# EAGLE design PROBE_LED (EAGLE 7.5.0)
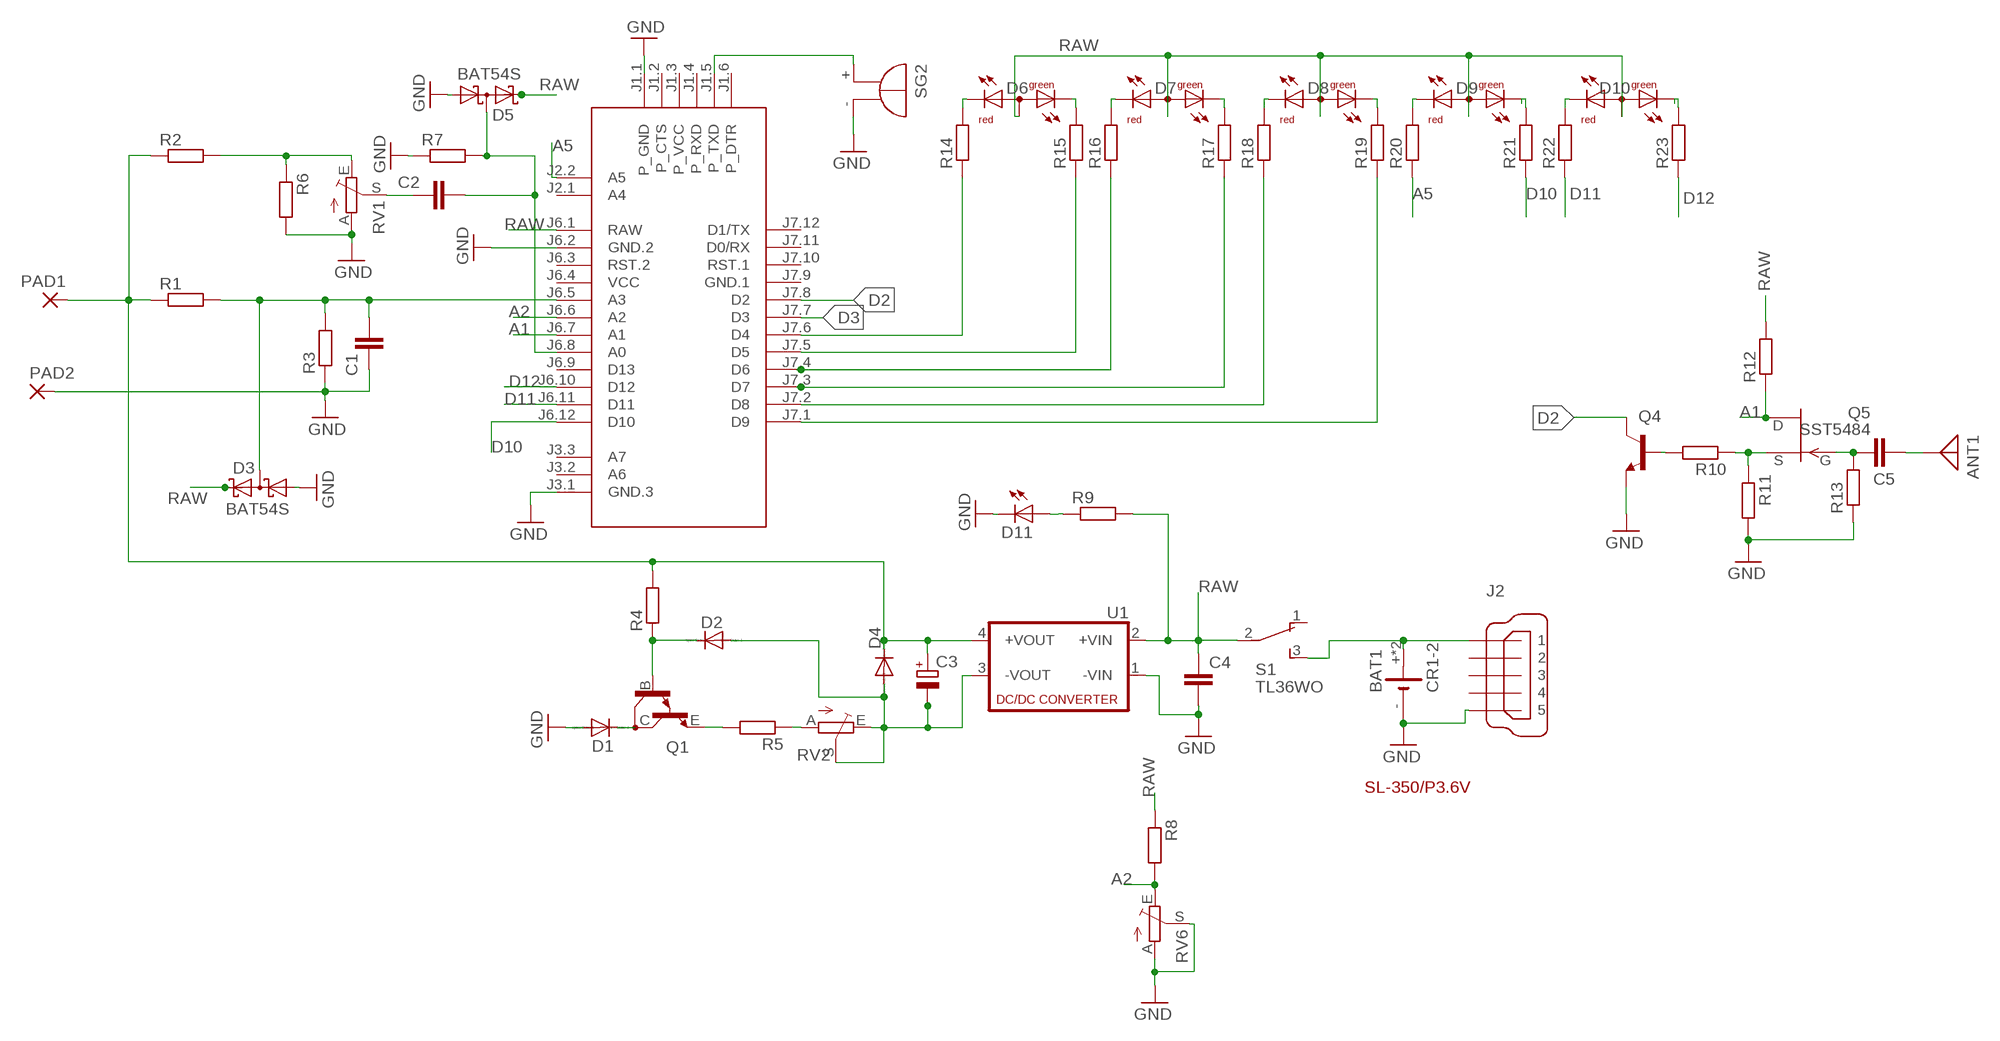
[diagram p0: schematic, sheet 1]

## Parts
ANT1  ANTENNA  [PAD-01]
ARD1  ARDUINO-PRO-MINI-3.3V  [ARDUINO-PRO-MINI]
BAT1  CR1-2  [CR1-2]
C1  C-EUC1206  [C1206]
C2  C-EUC1206  [C1206]
C3  CPOL-EUC/6032-28R  [C/6032-28R]
C4  C-EUC1206  [C1206]
C5  C-EUC1206  [C1206]
D1  CGRM4007-G  [SOD-123_MINI-SMA]
D2  CGRM4007-G  [SOD-123_MINI-SMA]
D3  BAT54S  [SOT23]
D4  CGRM4001-G  [SOD-123_MINI-SMA]
D5  BAT54S  [SOT23]
D6  DUOLED-RG-A  [DUOLED-A-5MM]
D7  DUOLED-RG-A  [DUOLED-A-5MM]
D8  DUOLED-RG-A  [DUOLED-A-5MM]
D9  DUOLED-RG-A  [DUOLED-A-5MM]
D10  DUOLED-RG-A  [DUOLED-A-5MM]
D11  LED5MM  [LED5MM]
J2  MINI-USB_SHIELD5P2-32005-601  [32005-601]
PAD1  3,81/1,1  [3,81/1,1]
PAD2  3,81/1,1  [3,81/1,1]
Q1  BDV65  [SOT93]
Q4  BC817-16LT1SMD  [SOT23-BEC]
Q5  SST5484  [SOT23]
R1  R-EU_R2512  [R2512]
R2  R-EU_R2512  [R2512]
R3  R-EU_R2512  [R2512]
R4  R-EU_R2512  [R2512]
R5  R-EU_R2512  [R2512]
R6  R-EU_R2512  [R2512]
R7  R-EU_R0805  [R0805]
R8  R-EU_R0805  [R0805]
R9  R-EU_R0805  [R0805]
R10  R-EU_R0805  [R0805]
R11  R-EU_R0805  [R0805]
R12  R-EU_R1206  [R1206]
R13  R-EU_R0805  [R0805]
R14  R-EU_R0805  [R0805]
R15  R-EU_R0805  [R0805]
R16  R-EU_R0805  [R0805]
R17  R-EU_R0805  [R0805]
R18  R-EU_R0805  [R0805]
R19  R-EU_R0805  [R0805]
R20  R-EU_R0805  [R0805]
R21  R-EU_R0805  [R0805]
R22  R-EU_R0805  [R0805]
R23  R-EU_R0805  [R0805]
RV1  TRIM_EU-CT6  [CT6]
RV2  TRIM_EU-CT6  [CT6]
RV6  TRIM_EU-CT6  [CT6]
S1  TL36WO  [TL3XWO]
SG2  BMT1205XH7.5  [BMT1205XH7.5]
U1  NME  [NME]

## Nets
A1: ARD1.J6.7(A1) Q5.2(D) R12.1
A2: ARD1.J6.6(A2) R8.2 RV6.E
A3: ARD1.J6.5(A3) C1.2 D3.3(C1A2) R1.2 R3.2
A5: ARD1.J2.2(A5) R20.1
D2: ARD1.J7.8(D2) Q4.C
D3: ARD1.J7.7(D3)
D10: ARD1.J6.12(D10) R21.1
D11: ARD1.J6.11(D11) R22.1
D12: ARD1.J6.10(D12) R23.1
GND: ARD1.J1.1(P_GND) ARD1.J3.1(GND.3) ARD1.J6.2(GND.2) BAT1.- C1.1 C4.2 D1.A D3.1(A1) D5.1(A1) D11.K(C) J2.5 PAD2.1(P) Q4.E R3.1 R6.2 R7.1 R11.2 R13.1 RV1.A RV6.A RV6.S SG2.- U1.1(-VIN)
N$1: R2.2 R6.1 RV1.E
N$2: Q4.B R10.2
N$3: Q5.3(S) R10.1 R11.1
N$4: ARD1.J6.8(A0) C2.2 D5.3(C1A2) R7.2
N$5: ARD1.J1.5(P_TXD) SG2.+
N$6: BAT1.+ BAT1.+@1(+) J2.1 S1.3(S)
N$7: ANT1.1 C5.2
N$8: Q1.E R5.2
N$9: R5.1 RV2.A
N$10: C3.- D2.A D4.A RV2.E RV2.S U1.3(-VOUT)
N$11: D6.CR R14.2
N$12: D1.C Q1.C
N$13: C5.1 Q5.1(G) R13.2
N$14: D6.CX(CG) R15.2
N$15: D7.CR R16.2
N$16: D7.CX(CG) R17.2
N$17: D8.CR R18.2
N$18: D8.CX(CG) R19.2
N$19: D9.CR R20.2
N$20: D2.C Q1.B R4.1
N$21: D9.CX(CG) R21.2
N$22: D10.CR R22.2
N$23: C2.1 RV1.S
N$24: C3.+ D4.C PAD1.1(P) R1.1 R2.1 R4.2 U1.4(+VOUT)
N$25: D10.CX(CG) R23.2
N$26: ARD1.J7.6(D4) R14.1
N$27: ARD1.J7.5(D5) R15.1
N$28: ARD1.J7.4(D6) R16.1
N$29: ARD1.J7.3(D7) R17.1
N$30: ARD1.J7.2(D8) R18.1
N$31: ARD1.J7.1(D9) R19.1
N$32: D11.A R9.1
RAW: ARD1.J6.1(RAW) C4.1 D3.2(C2) D5.2(C2) D6.A D7.A D8.A D9.A D10.A R8.1 R9.2 R12.2 S1.2(P) U1.2(+VIN)
Unconnected: ARD1.J1.2(P_CTS) ARD1.J1.3(P_VCC) ARD1.J1.4(P_RXD) ARD1.J1.6(P_DTR) ARD1.J2.1(A4) ARD1.J3.2(A6) ARD1.J3.3(A7) ARD1.J6.3(RST.2) ARD1.J6.9(D13) ARD1.J7.10(RST.1) ARD1.J7.11(D0/RX) ARD1.J7.12(D1/TX) J2.2 J2.3 J2.4 J2.M1(S1) J2.M2(S2) S1.1(O)

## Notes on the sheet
- SL-350/P3.6V

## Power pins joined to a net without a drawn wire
GND.1: ARD1.J7.9(GND.1)
VCC: ARD1.J6.4(VCC)

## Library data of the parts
ANT1 = discrete:ANTENNA: Antenna
ARD1 = diy-modules:ARDUINO-PRO-MINI-*: Arduino Pro Mini and compatible devices More details available here: https://www.arduino.cc/en/Main/ArduinoBoardProMini Click here to find device on ebay.com
BAT1 = battery:CR1-2
C1 C2 C4 C5 = rcl:C-EU: CAPACITOR, European symbol
C3 = rcl:CPOL-EU: POLARIZED CAPACITOR, European symbol
D1 D2 D4 = diode:CGRM400*-G: Molded plasitc,JEDEC SOD-123/Mini SMA
D3 D5 = diode:BAT54S: Schottky Diodes Pin connection corrected 2011-05-04 Source: Fairchild .. BAT54.pdf
D6-D10 = led:DUOLED-RG-A: DUO LED 2 colors (red/green), 5 mm, round, common Anode www.ligitek.com or other producers.
D11 = led:LED: LED
J2 = con-cypressindustries:MINI-USB_SHIELD5P2-: MINI USB-B R/A DIP 5pol. Source: www.cypressindustries.com; OC_FARNELL: unknown; OC_NEWARK: unknown
PAD1 PAD2 = wirepad:3,81/1,1: THROUGH-HOLE PAD
Q1 = transistor:BDV65: NPN BIPOLAR DARLINGTON TRANSISTOR
Q4 = transistor-npn:BC817*: NPN Transistor
Q5 = transistor-fet:?548*: N-Channel JFETs Source: VISHAY 2N5484.pdf Compatible: TO92 2N5245 J304 J305 U310 J308 J309 J310 TO72 2N4416 2N4416A 2N3823 2N4351 3N169 3N170 3N171 MFE3002 TO18 2N3796 2N3797 MFE825 Source: Motorola European Master Guide Pacge 3-59
R1-R23 = rcl:R-EU_: RESISTOR, European symbol
RV1 RV2 RV6 = pot:TRIM_EU-: POTENTIOMETER
S1 = switch:TL36WO: TINY SWITCH ON - ON Source: http://www2.produktinfo.conrad.com/datenblaetter/700000-724999/705152-da-01-de-Subminiaturschalter_TL_36WO.pdf
SG2 = buzzer:BMT1205XH7.5: MAGNETIC TRANSDUCER; OC_FARNELL: unknown; OC_NEWARK: unknown
U1 = dc-dc-converter:NME: DC-DC CONVERTER; MF: C & D TECHNOLOGIES, INC; MPN: NME1205D; OC_FARNELL: 1021466; OC_NEWARK: 98B8198

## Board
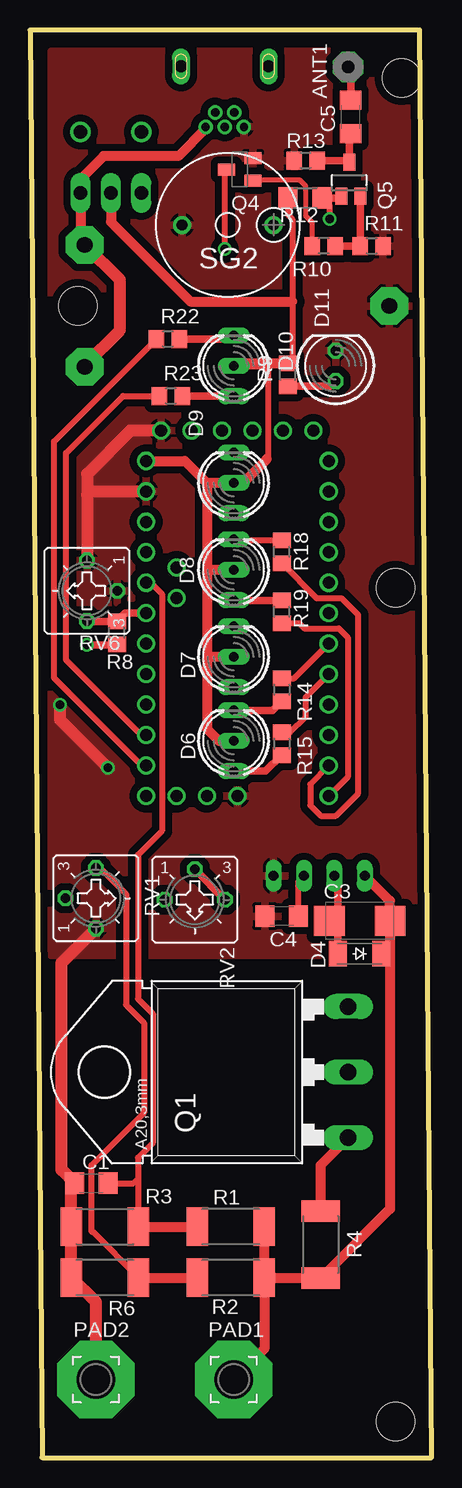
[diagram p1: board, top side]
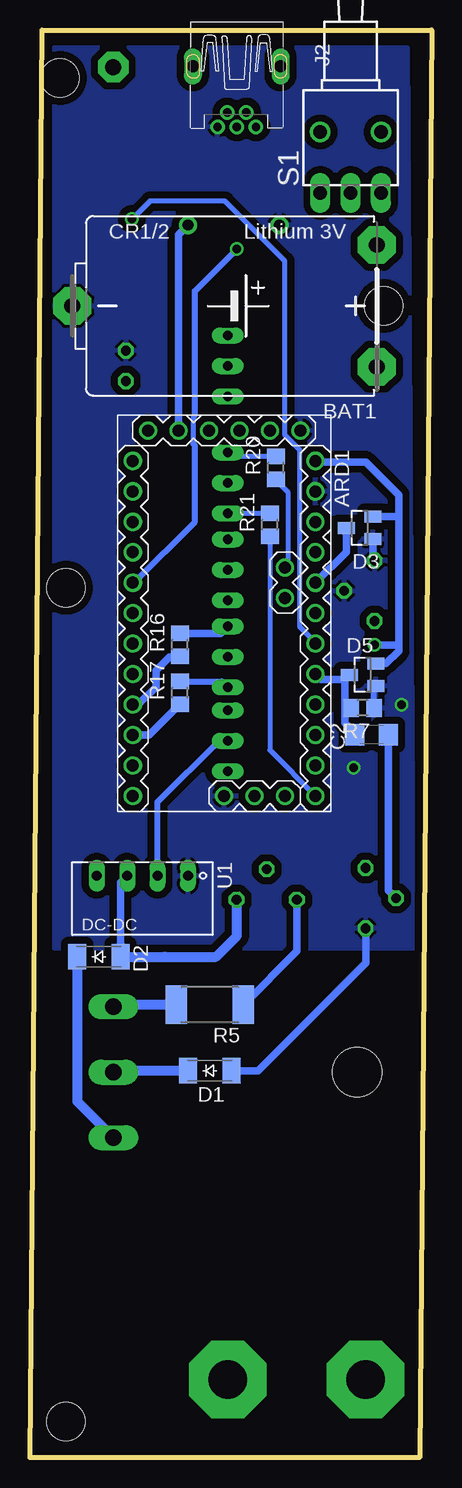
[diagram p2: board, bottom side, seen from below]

Size 33.5 x 119 mm. Coordinates in mm from the lower left corner, seen from the top.
Outline: 1,0 33.5,0 32.5,119 0,119 1,0
Copper layers (1*16): Top 0.035mm / dielectric 1.5mm / Bottom 0.035mm
Design rules "default *": minimum track width 10mil, minimum drill 24mil, track to track 8mil, track to pad 8mil, pad to pad 8mil, via to via 8mil, smd to smd 8mil, copper to edge 20mil, drill to drill 8mil, minimum pad ring 10mil, minimum via ring 8mil, stop-mask expansion 4mil, vias tented up to drill 0mil, thermal gap 10mil
Holes 3.2 mm at 31,115 30.5,3 30.5,72.5 4,96
bRestrict: area 1.4,22.6 to 11,28.2

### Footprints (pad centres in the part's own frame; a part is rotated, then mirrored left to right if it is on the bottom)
PAD-01 = drill 1.321 pad 2.54 octagon: 1 0,0
ARDUINO-PRO-MINI = drill 1: J1.1 -15.24,6.35; J1.2 -15.24,3.81; J1.3 -15.24,1.27; J1.4 -15.24,-1.27; J1.5 -15.24,-3.81; J1.6 -15.24,-6.35; J2.1 -1.27,5.08; J2.2 -3.81,5.08; J3.1 15.24,0; J3.2 15.24,2.54; J3.3 15.24,5.08; J6.1 -12.7,7.62; J6.2 -10.16,7.62; J6.3 -7.62,7.62; J6.4 -5.08,7.62; J6.5 -2.54,7.62; J6.6 0,7.62; J6.7 2.54,7.62; J6.8 5.08,7.62; J6.9 7.62,7.62; J6.10 10.16,7.62; J6.11 12.7,7.62; J6.12 15.24,7.62; J7.1 15.24,-7.62; J7.2 12.7,-7.62; J7.3 10.16,-7.62; J7.4 7.62,-7.62; J7.5 5.08,-7.62; J7.6 2.54,-7.62; J7.7 0,-7.62; J7.8 -2.54,-7.62; J7.9 -5.08,-7.62; J7.10 -7.62,-7.62; J7.11 -10.16,-7.62; J7.12 -12.7,-7.62
CR1-2 = drill 1.321 pad 3.15 octagon: + -11.43,-5.08; +@1 -11.43,5.08; - 13.97,0
C1206 = smd 1.6 x 1.8: 1 -1.4,0; 2 1.4,0
C/6032-28R = smd 2.55 x 2.5: + 2.525,0; - -2.525,0
SOD-123_MINI-SMA = smd 1.5 x 2.1: A 1.8,0; C -1.8,0
SOT23 = smd 1 x 1.4: 1 -0.95,-1.1; 2 0.95,-1.1; 3 0,1.1
DUOLED-A-5MM = drill 0.813 long: A 0,0; CR 2.54,0; CX -2.54,0
LED5MM = drill 0.813 octagon: A -1.27,0; K 1.27,0
32005-601 = drill 0.7 pad 1.016: 1 2.825,1.6; 2 1.625,0.8; 3 2.825,0; 4 1.625,-0.8; 5 2.825,-1.6 | drill 1 pad 1.422 long: M1 -2.225,3.65; M2 -2.225,-3.65
3,81/1,1 = drill 3.2 pad 6.452 octagon: 1 0,0
SOT93 = drill 1.397 long: B -5.461,-10.16; C 0,-10.16; E 5.461,-10.16 | hole 4.115: 0,10.16
SOT23-BEC = smd 1 x 1.4: B -0.95,-1.1; C 0,1.1; E 0.95,-1.1
SOT23' = smd 1 x 1.4: 1 0,1.735; 2 -0.632,-1.1; 3 0.95,-1.1
R2512 = smd 1.8 x 3.2: 1 -2.8,0; 2 2.8,0
R0805 = smd 1.3 x 1.5: 1 -0.95,0; 2 0.95,0
R1206 = smd 1.6 x 1.803: 1 -1.422,0; 2 1.422,0
CT6 = drill 0.813 octagon: A 2.515,0; E -2.515,0; S 0,-2.54
TL3XWO = drill 1.1 pad 1.422 long: 1 -2.54,-5.08; 2 0,-5.08; 3 2.54,-5.08 | drill 1.1 pad 1.676: M1 -2.54,0; M2 2.54,0
BMT1205XH7.5 = drill 0.9 pad 1.5: + 3.8,0; - -3.8,0
NME = drill 0.813 long: 1 0,3.81; 2 0,1.27; 3 0,-1.27; 4 0,-3.81

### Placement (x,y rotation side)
ANT1  26.55,115.91 0 top
ARD1  17.3,70.38 270 bottom
BAT1  16,96 180 bottom
C1  5.12,22.88 0 top
C2  5,60.25 180 bottom
C3  27.5,44.75 0 top
C4  21,45.12 180 top
C5  26.75,111.75 90 top
D1  18.5,32.25 0 bottom
D2  27.75,41.75 0 bottom
D3  6,77.5 90 bottom
D4  27.5,42 180 top
D5  5.75,65.25 90 bottom
D6  17,59.75 90 top
D7  17,66.75 90 top
D8  17,74 90 top
D9  17,81.25 90 top
D10  17,91 90 top
D11  25.5,91 90 top
J2  16.25,113.75 270 bottom
PAD1  17,6.5 0 top
PAD2  5.5,6.5 0 top
Q1  16.38,32.12 90 top
Q4  17.5,107.38 90 top
Q5  SST5484  [SOT23']  26.62,106.25 0 top
R1  16.75,19.25 180 top
R2  16.75,15 180 top
R3  6.25,19.25 0 top
R4  24.25,17.75 270 top
R5  18.5,37.75 180 bottom
R6  6.25,15 180 top
R7  5.75,62.5 180 bottom
R8  7.25,68.75 90 top
R9  21.5,90.25 90 top
R10  24.5,101 180 top
R11  28.5,101 0 top
R12  22.95,105 180 top
R13  23,108.12 0 top
R14  21,64 270 top
R15  21,59.5 270 top
R16  21,67.75 90 bottom
R17  21,63.75 90 bottom
R18  21,75.5 90 top
R19  21,70.5 90 top
R20  13,82.5 90 bottom
R21  13.5,77.75 90 bottom
R22  11.5,93.25 0 top
R23  11.75,88.5 0 top
RV1  5.5,46.62 270 top
RV2  13.75,46.5 180 top
RV6  4.75,72.25 90 top
S1  6.75,110.5 0 bottom
SG2  16.5,102.75 0 top
U1  24.12,48.5 270 bottom

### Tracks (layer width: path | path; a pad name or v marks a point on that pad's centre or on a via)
A1  (via drill 0.7)
  Top 0.406: 24.5,104.87 R12.1
  Top 0.5: v25,103.25 25,104.37 R12.1
  Top 0.61: R12.1 25.84,105 Q5.2
  Bottom 0.406: ARD1.J6.7 9.68,67.93 11,69.25 11,84 12.25,85.25 12.25,99.75 17.25,104.75 23.5,104.75 v25,103.25
A2
  Top 0.61: RV6.E 4.79,69.7 R8.2 7.93,70.38 ARD1.J6.6
A3
  Top 0.5: 9,23.25 9,25 10.25,26.25 10.25,37 9,38.25 9,50.25 11,52.25 11,72 10.08,72.92 ARD1.J6.5 | 9,23.25 9,19.3 R3.2 | C1.2 8.62,22.88 9,23.25
  Top 0.813: R3.2 R1.2
  Bottom 0.61: D3.3 7.1,75.5 ARD1.J6.5
A5
  Bottom 0.406: R20.1 13,81.5 12,80.5 12,74.41 ARD1.J2.2
D2  (via drill 0.7)
  Top 0.5: v16.25,100.75 16.25,107.22 Q4.C
  Bottom 0.406: 19.88,84.5 19.88,86.75 19.75,86.88
  Bottom 0.5: ARD1.J7.8 24.83,72.92 19.75,78 19.75,84.38 19.88,84.5 | v16.25,100.75 19.75,97.25 19.75,86.88
D10
  Bottom 0.406: R21.1 13.5,58.96 ARD1.J6.12
D11
  Top 0.5: ARD1.J6.11 9.32,57.68 2,65 2,84.7 R22.1
D12
  Top 0.5: ARD1.J6.10 9.28,60.22 3,66.5 3,83.75 7.75,88.5 R23.1
GND  (via drill 0.7)
  Top 1.016: RV1.A 2.62,41.23 2.62,23.98 C1.1 3.45,22.6 R3.1 R6.2 5.5,12.95 PAD2.1 | v6.5,57.5 2.5,61.5 v2.5,62.75 | ARD1.J1.1 8.37,85.62 4.75,82 4.75,80.25 | 4.75,80.25 RV6.A | ARD1.J6.2 5.04,80.54 4.75,80.25
  Bottom 0.5: R7.1 4.8,64.15 D5.1
  Bottom 0.61: D3.1 4.9,74.92 RV6.A | D1.A 14.5,32.25 5.5,41.25 RV1.A
  pour Bottom (isolate 0.61): 2,117.5 31.5,117.5 31.5,42.5 1.5,42.5
  pour Top (isolate 0.61): 1.75,117.25 33.12,117.25 33.12,41.88 1.75,41.88
N$1
  Top 0.5: RV1.E 5.86,49.14 8,47 8,37.75 9.5,36.25 9.5,28.75 5.12,24.38 5.12,18.88 5.2,18.8 5.25,18.8 R6.1
  Top 0.813: R6.1 R2.2
N$2
  Top 0.406: R10.2 23.55,102.95 23,103.5 23,106 22.5,106.5 18.68,106.5 Q4.B
N$3
  Top 0.61: R10.1 R11.1 27.55,105.12 Q5.3
N$4
  Bottom 0.5: R7.2 6.75,62.5 7.25,63
  Bottom 0.61: C2.2 6.4,60.4 7.25,61.25 7.25,63 7.25,64.85 | 7.25,64.85 D5.3 | 7.25,64.85 9.23,64.85 ARD1.J6.8
N$5
  Bottom 0.61: ARD1.J1.5 21.11,101.94 SG2.+
N$6
  Top 0.813: BAT1.+ 4.21,101.44 S1.3 4.12,105.5 4.12,106.5 6.12,108.5 12.38,108.5 14.65,110.78 J2.1
  Top 1.016: BAT1.+@1 4.57,91.07 7.5,94 7.5,98.15 BAT1.+
N$7
  Top 0.61: C5.2 26.75,115.71 ANT1.1
N$8
  Bottom 0.813: R5.2 26.37,37.75 Q1.E
N$9
  Bottom 0.61: RV2.A 11.23,42.22 R5.1
N$10
  Top 0.61: 25,44.5 24.98,44.52 C3.- 25.7,44.02 D4.A 25.7,48.2 U1.3 | RV2.S 13.75,49.02 RV2.E
  Bottom 0.61: D2.A 25.95,47.95 U1.3
  Bottom 0.813: D2.A 22.25,41.75 18,41.75 16.25,43.5 16.25,46.48 RV2.E
N$11
  Top 0.61: D6.CR 20.24,62.29 R14.2
N$12
  Bottom 0.813: D1.C 26.41,32.25 Q1.C
N$13
  Top 0.61: Q5.1 26.62,108 | 26.62,108 26.62,110.22 C5.1 | R13.2 26.5,108.12 26.62,108
N$14
  Top 0.61: D6.CX 19.66,57.21 R15.2
N$15
  Bottom 0.61: R16.2 17.59,68.7 D7.CR
N$16
  Bottom 0.5: R17.2 17.49,64.7 D7.CX
N$17
  Top 0.5: R18.2 17.09,76.45 D8.CR
N$18
  Top 0.61: R19.2 D8.CX
N$19
  Bottom 0.406: R20.2 16.66,83.45 D9.CR
N$20
  Top 0.813: R4.1 24.25,24.38 Q1.B
  Bottom 0.813: D2.C 29.55,29.68 Q1.B
N$21
  Bottom 0.406: R21.2 D9.CX
N$22
  Top 0.61: R22.2 16.71,93.25 D10.CR
N$23
  Bottom 0.61: C2.1 3.6,47.27 RV1.S
N$24
  Top 0.813: R2.1 19.55,9.05 PAD1.1 | R2.1 24.2,15 R4.2 30.02,20.73 30.02,42 | R2.1 R1.1 | 30.02,42 C3.+ 30.02,46.41 U1.4 | D4.C 30.02,42
N$25
  Top 0.61: R23.2 16.96,88.5 D10.CX
N$26
  Top 0.5: R14.1 22.03,64.95 ARD1.J7.6
N$27
  Top 0.5: R15.1 21.7,60.45 23,61.75 23,63.38 ARD1.J7.5
N$28
  Bottom 0.61: ARD1.J7.4 24.49,62.76 23,64.25 23,65.62 21.88,66.75 21.05,66.75 R16.1
N$29
  Bottom 0.61: ARD1.J7.3 23.58,60.22 R17.1
N$30
  Top 0.5: ARD1.J7.2 23.38,56.12 23.38,54.38 24.25,53.5 25.5,53.5 27.38,55.38 27.38,70.25 26,71.62 23.93,71.62 R18.1
N$31
  Top 0.5: R19.1 22.45,69.55 22.88,69.12 25.75,69.12 26.5,68.38 26.5,56.72 ARD1.J7.1
N$32
  Top 0.61: R9.1 25.07,89.3 D11.A
RAW  (via drill 0.7)
  Top 0.5: C4.1 22.4,48.05 U1.2 | D10.A 19.75,91 19.88,90.88 19.88,83.38 19.75,83.25 | R12.2 21.53,103.6 21.88,103.25 21.88,96.38 21.88,91.58 R9.2
  Top 0.61: v4.75,67.75 7.2,67.75 R8.1
  Top 0.813: R9.2 17.2,91.2 D10.A | 19.75,83.25 17.75,81.25 D9.A 15,81.25 14.75,81 | ARD1.J6.1 12.92,83.08 14.75,81.25 14.75,81 | 14.75,81 14.75,73.75 | 14.75,73.75 14.75,66.5 | 14.75,66.5 14.75,60.75 15.75,59.75 D6.A | D7.A 15,66.75 14.75,66.5 | D8.A 15,74 14.75,73.75 | S1.2 6.75,103 13.38,96.38 21.88,96.38
  Bottom 0.5: U1.2 22.86,54.65 17.75,59.75 D6.A
  Bottom 0.61: D5.2 3.8,66.2 2.75,67.25 2.75,67.75 | 2.75,67.75 2.75,78.25 | 2.75,78.25 2.75,80.25 5.5,83 9.6,83 ARD1.J6.1 | D3.2 2.95,78.45 2.75,78.25 | v4.75,67.75 2.75,67.75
